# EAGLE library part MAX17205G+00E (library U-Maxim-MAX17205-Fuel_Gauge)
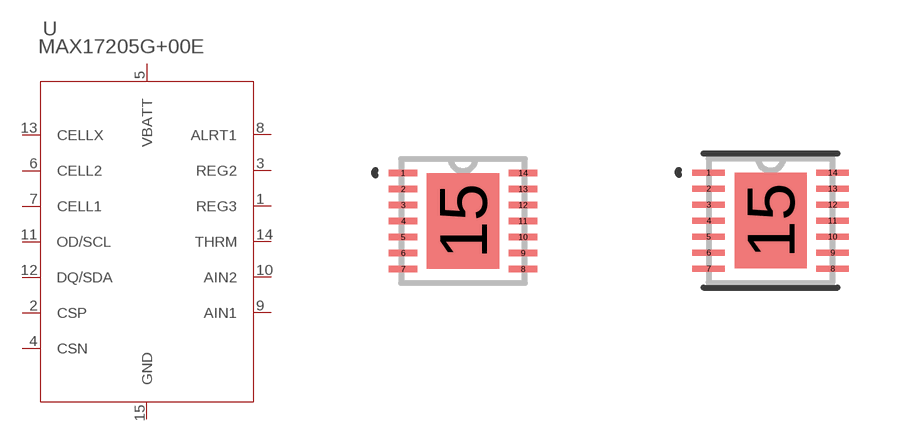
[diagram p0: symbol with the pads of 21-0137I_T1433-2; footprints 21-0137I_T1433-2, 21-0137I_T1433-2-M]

Designator prefix U

## MAX17205G+00E (MANUFACTURER_PART_NUMBER: MAX17205G+00E; VENDOR: Maxim Integrated Products)  [21-0137I_T1433-2]
1  REG3
2  CSP  pas
3  REG2
4  CSN  pas
5  VBATT  pas
6  CELL2
7  CELL1
8  ALRT1  pas
9  AIN1  in
10  AIN2  in
11  OD/SCL  pas
12  DQ/SDA  pas
13  CELLX  pas
14  THRM  pas
15  GND  pas

## MAX17205G+00E21-0137I_T1433-2-M (MANUFACTURER_PART_NUMBER: MAX17205G+00E; VENDOR: Maxim Integrated Products)  [21-0137I_T1433-2-M]
Pads as for 21-0137I_T1433-2

## MAX17205G+00E21-0137I_T1433-2-L (MANUFACTURER_PART_NUMBER: MAX17205G+00E; VENDOR: Maxim Integrated Products)  [21-0137I_T1433-2-L]
Pads as for 21-0137I_T1433-2

## Footprint 21-0137I_T1433-2 (pad centres in mm)
smd 0.711 x 0.152: 1 -1.499,1.2; 2 -1.499,0.8; 3 -1.499,0.4; 4 -1.499,0; 5 -1.499,-0.4; 6 -1.499,-0.8; 7 -1.499,-1.2; 8 1.499,-1.2; 9 1.499,-0.8; 10 1.499,-0.4; 11 1.499,0; 12 1.499,0.4; 13 1.499,0.8; 14 1.499,1.2
smd 1.803 x 2.388: 15 0,0

## Footprint 21-0137I_T1433-2-M (pad centres in mm)
smd 0.813 x 0.152: 1 -1.549,1.2; 2 -1.549,0.8; 3 -1.549,0.4; 4 -1.549,0; 5 -1.549,-0.4; 6 -1.549,-0.8; 7 -1.549,-1.2; 8 1.549,-1.2; 9 1.549,-0.8; 10 1.549,-0.4; 11 1.549,0; 12 1.549,0.4; 13 1.549,0.8; 14 1.549,1.2
smd 1.803 x 2.388: 15 0,0

## Footprint 21-0137I_T1433-2-L (pad centres in mm)
smd 0.61 x 0.152: 1 -1.448,1.2; 2 -1.448,0.8; 3 -1.448,0.4; 4 -1.448,0; 5 -1.448,-0.4; 6 -1.448,-0.8; 7 -1.448,-1.2; 8 1.448,-1.2; 9 1.448,-0.8; 10 1.448,-0.4; 11 1.448,0; 12 1.448,0.4; 13 1.448,0.8; 14 1.448,1.2
smd 1.803 x 2.388: 15 0,0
